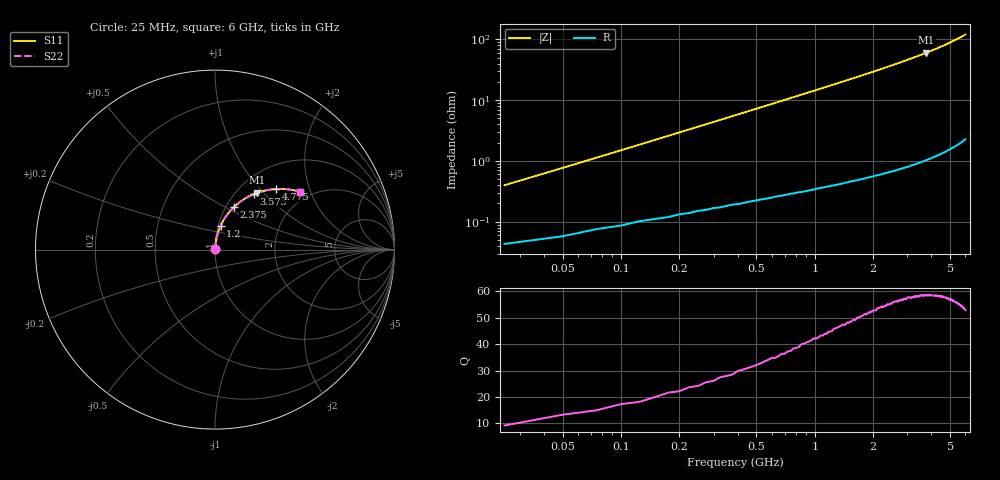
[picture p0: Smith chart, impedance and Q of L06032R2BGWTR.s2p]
!	AVX Thin Film Operation
!	Date:	March	2003
!	Description: Accu-L® Series Thin Film SMD RF Inductors
!	Part Number: L06032R2BGWTR
!	25MHz-6GHz
!	Serial	Measurements
#	mhz	S	db	R	50
!	S11	S11	S21	S21	S12	S12	S22	S22
!	dB	Phase	dB	Phase	dB	Phase	dB	Phase
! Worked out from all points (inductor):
!   240 points, 25 MHz to 6 GHz, reference 50 ohm
!   read as 1/Y11, port 2 shorted: L = 2.41 nH near 50 MHz
!   highest Q = 58.6 at 3.775 GHz (marker M1), where L = 2.55 nH
!   S11 on the Smith chart (normalised r, x): 25 MHz: 1.00, +0.01; 1.2 GHz: 1.03, +0.28; 2.375 GHz: 1.09, +0.56; 3.575 GHz: 1.21, +0.87; 4.775 GHz: 1.41, +1.24; 6 GHz: 1.76, +1.69
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25  -49.65 82.6  -0.00 -0.3  -0.00 -0.3  -49.65 82.6
50  -44.00 84.0  -0.01 -0.5  -0.01 -0.5  -44.00 84.0
75  -40.66 84.6  -0.01 -0.8  -0.01 -0.8  -40.66 84.6
100  -38.27 84.8  -0.01 -1.0  -0.01 -1.0  -38.27 84.8
125  -36.41 84.9  -0.01 -1.3  -0.01 -1.3  -36.41 84.9
175  -33.59 84.9  -0.01 -1.8  -0.01 -1.8  -33.59 84.9
275  -29.78 84.5  -0.02 -2.7  -0.02 -2.7  -29.78 84.5
400  -26.62 83.6  -0.03 -4.0  -0.03 -4.0  -26.62 83.6
575  -23.54 82.2  -0.04 -5.7  -0.04 -5.7  -23.54 82.2
775  -21.02 80.5  -0.06 -7.6  -0.06 -7.6  -21.02 80.5
1025  -18.65 78.3  -0.09 -10.0  -0.09 -10.0  -18.65 78.3
1200  -17.32 76.7  -0.11 -11.7  -0.11 -11.7  -17.32 76.7
1575  -15.05 73.2  -0.17 -15.3  -0.17 -15.3  -15.05 73.2
2025  -12.97 69.1  -0.27 -19.5  -0.27 -19.5  -12.97 69.1
2375  -11.67 65.9  -0.35 -22.8  -0.35 -22.8  -11.67 65.9
3025  -9.75 60.0  -0.54 -28.8  -0.54 -28.8  -9.75 60.0
3575  -8.46 55.0  -0.73 -33.7  -0.73 -33.7  -8.46 55.0
3775  -8.05 53.2  -0.80 -35.5  -0.80 -35.5  -8.05 53.2
4025  -7.58 51.0  -0.90 -37.7  -0.90 -37.7  -7.58 51.0
4775  -6.36 44.6  -1.22 -44.2  -1.22 -44.2  -6.36 44.6
5025  -6.01 42.5  -1.33 -46.3  -1.33 -46.3  -6.01 42.5
6000  -4.85 34.4  -1.81 -54.3  -1.81 -54.3  -4.85 34.4
